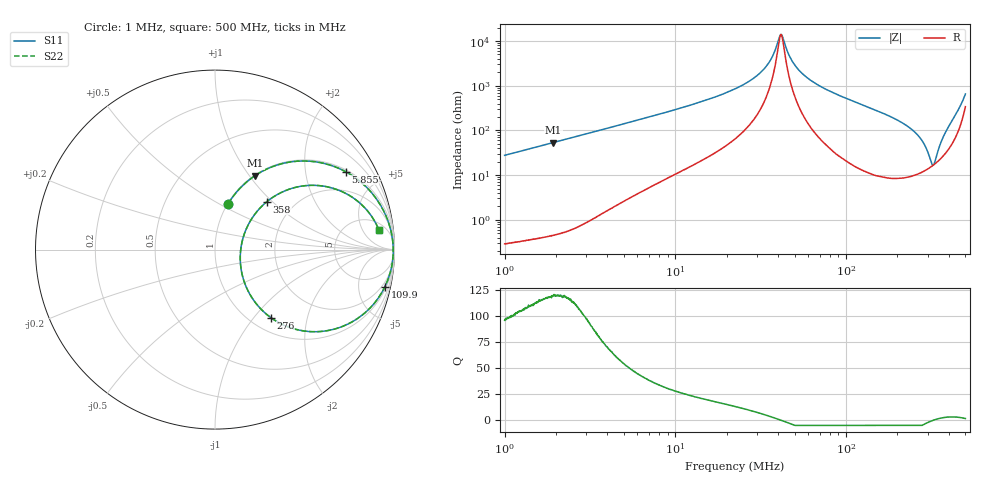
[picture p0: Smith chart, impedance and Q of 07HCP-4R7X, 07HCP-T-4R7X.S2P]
!s-Parameter Generated by FASTRON Sdn. Bhd.
!FASTRON P/N : 07HCP-4R7X, 07HCP/T-4R7X
!Keysight Technologies,E4991B,MY54100416,A.01.15
!Date: Fri Feb 20 12:48:45 2026
!Version  : Rev00 Fri Feb 20 12:48:45 2026
!Data & Calibration Information:
!PortZ  Port1:50+j0  Port2:50+j0
!When reading, reference impedance value at option line is always used.
! Remarks : This data is being provided solely for informational purposes.
!Freq	S11	S21	S12	S22
# Hz S dB R 50
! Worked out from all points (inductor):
!   1601 points, 1 MHz to 500 MHz, reference 50 ohm
!   read as one part in series: L = 4.4 uH near 1.032 MHz
!   highest Q = 119 at 1.928 MHz (marker M1), where L = 4.41 uH
!   self-resonance near 41.47 MHz
!   S11 on the Smith chart (normalised r, x): 1 MHz: 1.01, +0.55; 5.855 MHz: 1.07, +3.31; 109.9 MHz: 1.33, -9.03; 276 MHz: 1.23, -1.23; 358 MHz: 1.47, +0.93; 500 MHz: 8, +11
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1000000  -11.49 74.0  -0.34 -15.4  -0.34 -15.4  -11.49 74.0
1927874  -6.57 61.5  -1.12 -28.0  -1.12 -28.0  -6.57 61.5
2820919  -4.23 51.5  -2.12 -37.9  -2.12 -37.9  -4.23 51.5
5854902  -1.44 30.8  -5.80 -57.9  -5.80 -57.9  -1.44 30.8
7957584  -0.86 23.4  -8.01 -64.9  -8.01 -64.9  -0.86 23.4
2.236068e7  -0.14 6.6  -18.71 -79.0  -18.71 -79.0  -0.14 6.6
2.822906e7  -0.09 4.0  -23.01 -79.5  -23.01 -79.5  -0.09 4.0
3.323107e7  -0.07 2.3  -27.76 -77.1  -27.76 -77.1  -0.07 2.3
3.661978e7  -0.07 1.3  -32.41 -71.0  -32.41 -71.0  -0.07 1.3
4.162766e7  -0.06 -0.0  -43.00 1.1  -43.00 1.1  -0.06 -0.0
4.957817e7  -0.06 -1.8  -29.77 76.1  -29.77 76.1  -0.06 -1.8
6.307767e7  -0.08 -4.5  -22.13 80.7  -22.13 80.7  -0.08 -4.5
1.099249e8  -0.27 -12.4  -13.37 75.5  -13.37 75.5  -0.27 -12.4
1.77937e8  -1.00 -24.8  -7.54 62.9  -7.54 62.9  -1.00 -24.8
2.36269e8  -2.81 -39.2  -3.95 46.1  -3.95 46.1  -2.81 -39.2
2.759822e8  -6.19 -50.6  -2.09 28.8  -2.09 28.8  -6.19 -50.6
3.223705e8  -16.90 -8.4  -1.32 1.4  -1.32 1.4  -16.90 -8.4
3.312556e8  -15.48 22.1  -1.45 -4.3  -1.45 -4.3  -15.48 22.1
3.580143e8  -8.10 42.7  -2.39 -20.6  -2.39 -20.6  -8.10 42.7
4.053963e8  -2.98 29.7  -5.68 -42.5  -5.68 -42.5  -2.98 29.7
4.484748e8  -1.42 17.7  -9.88 -53.5  -9.88 -53.5  -1.42 17.7
5e8  -0.73 6.9  -17.03 -51.7  -17.03 -51.7  -0.73 6.9
